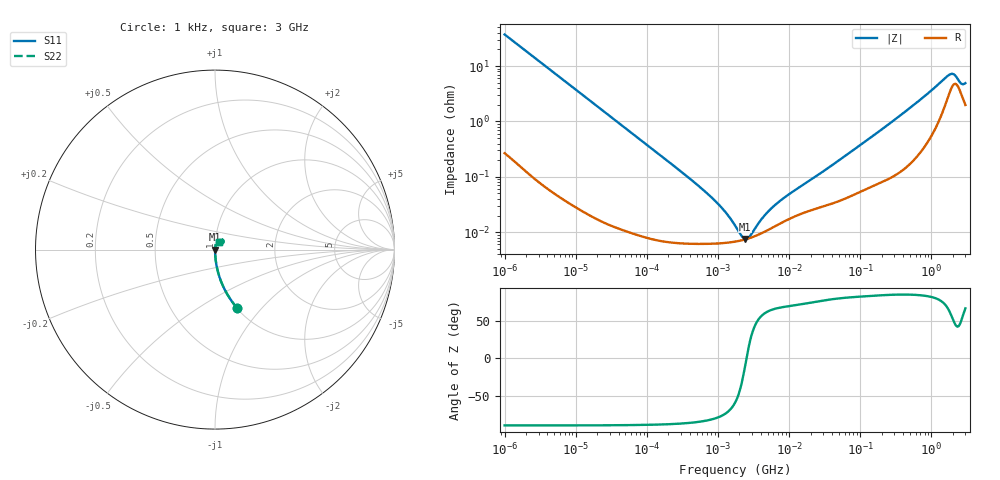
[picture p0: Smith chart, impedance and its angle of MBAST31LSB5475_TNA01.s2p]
! MBAST31LSB5475_TNA01  S-PARAMETER MODEL  ( Standard Model )
! Model Generated by TAIYO YUDEN Corporation (http://www.ty-top.com)
! Version 1.0
! TAIYO YUDEN Control No. 220601
! Copyright(c) 2012 TAIYO YUDEN CO.,LTD. All Rights Reserved.
! Product Description (link to TY-COMPAS)
! https://ds.yuden.co.jp/TYCOMPAS/or/detail?pn=MBAST31LSB5475KTNA01&u=M
! Products Name : Multilayer Ceramic Capacitors
! Characteristics :
!  Capacitance : 4.7 [uF] , Rated Voltage : 25 [V] , TCC : X5R
!  Case Size : 3.2 x 1.6 / 0.126 x 0.063 [mm/inch] , Thickness : 1.6 / 0.063 [mm/inch]
!  (Conditions: Temperature = 25 [degC] , DC Bias Voltage = 0 [V])
! External Node Assignments :
!  1  o---| |---o  2
! GND o---------o GND
! Frequency Range : 1kHz  -  3GHz  [ 401 STEP ]
# MHZ S RI R 50
! Freq[MHz].  S11 Real  S11 Imag  S21 Real  S21 Imag  S12 Real  S12 Imag  S22 Real  S22 Imag
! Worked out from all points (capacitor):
!   401 points, 1 kHz to 3 GHz, reference 50 ohm
!   read as one part in series: C = 4.26 uF near 1.077 kHz
!   lowest |Z| = 7.5 mohm at 2.423 MHz (marker M1)
!   series resonance near 2.517 MHz, so ESL is about 940 pH
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0.001  0.1239 -0.3259  0.8761 0.3259  0.8761 0.3259  0.1239 -0.3259
0.001685  0.0482 -0.2109  0.9518 0.2109  0.9518 0.2109  0.0482 -0.2109
0.00306  0.0155 -0.1205  0.9845 0.1205  0.9845 0.1205  0.0155 -0.1205
0.01216  0.0012 -0.0309  0.9988 0.0309  0.9988 0.0309  0.0012 -0.0309
0.147855  7.67e-05 -0.00256  0.9999 0.00256  0.9999 0.00256  7.67e-05 -0.00256
0.419985  6.24e-05 -0.000881  0.9999 0.000881  0.9999 0.000881  6.24e-05 -0.000881
0.791611  6.19e-05 -0.000433  0.9999 0.000433  0.9999 0.000433  6.19e-05 -0.000433
1.238299  6.39e-05 -0.000232  0.9999 0.000232  0.9999 0.000232  6.39e-05 -0.000232
1.732051  6.74e-05 -0.000114  0.9999 0.000114  0.9999 0.000114  6.74e-05 -0.000114
2.010629  6.99e-05 -6.74e-05  0.9999 6.74e-05  0.9999 6.74e-05  6.99e-05 -6.74e-05
2.422679  7.42e-05 -1.13e-05  0.9999 1.13e-05  0.9999 1.13e-05  7.42e-05 -1.13e-05
3.03007  8.13e-05 5.43e-05  0.9999 -5.43e-05  0.9999 -5.43e-05  8.13e-05 5.43e-05
4.566395  0.000103 0.000177  0.9999 -0.000177  0.9999 -0.000177  0.000103 0.000177
6.387174  0.000129 0.000285  0.9999 -0.000285  0.9999 -0.000285  0.000129 0.000285
9.625639  0.000169 0.000439  0.9998 -0.000439  0.9998 -0.000439  0.000169 0.000439
21.06097  0.000253 0.000885  0.9997 -0.000885  0.9997 -0.000885  0.000253 0.000885
256.0921  0.00101 0.00904  0.999 -0.00904  0.999 -0.00904  0.00101 0.00904
1056.143  0.00762 0.0377  0.9924 -0.0377  0.9924 -0.0377  0.00762 0.0377
1780.008  0.0345 0.058  0.9655 -0.058  0.9655 -0.058  0.0345 0.058
2066.299  0.0473 0.0485  0.9527 -0.0485  0.9527 -0.0485  0.0473 0.0485
2584.342  0.033 0.0342  0.967 -0.0342  0.967 -0.0342  0.033 0.0342
3000  0.0214 0.0433  0.9786 -0.0433  0.9786 -0.0433  0.0214 0.0433
